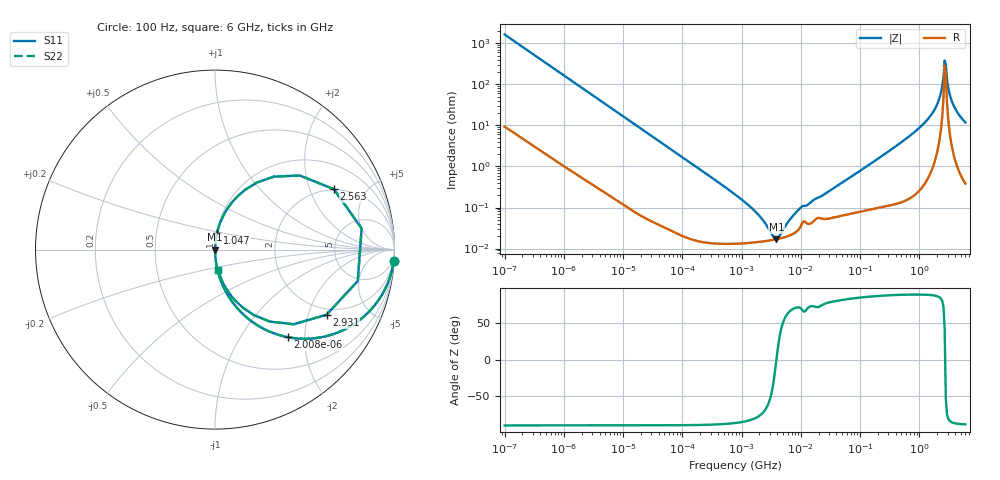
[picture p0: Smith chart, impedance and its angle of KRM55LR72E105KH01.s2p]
!Murata Part Number: KRM55LR72E105KH01
!These Parameters are Measured in Series Mode Connection
!Data Generated on Jan 08, 2026
!  o--ll--o
!Port1  Port2
!  o------o
!Operation Temp=25[degC], DC Bias Voltage=0[V]
!Freq. Start=100[Hz] Stop=6[GHz] 401[Steps]
# Hz S RI R 50
!Freq.(Hz) S11(Real) S11(Imag) S21(Real) S21(Imag) S12(Real) S12(Imag) S22(Real) S22(Imag)
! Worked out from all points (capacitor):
!   401 points, 100 Hz to 6 GHz, reference 50 ohm
!   read as one part in series: C = 972 nF near 109 Hz
!   lowest |Z| = 16.8 mohm at 3.882 MHz (marker M1)
!   series resonance near 3.878 MHz, so ESL is about 1.7 nH
!   S11 on the Smith chart (normalised r, x): 100 Hz: 1, -33; 2.008 kHz: 1.01, -1.65; 1.047 GHz: 1.01, +0.18; 2.563 GHz: 1.97, +2.96; 2.931 GHz: 1.75, -2.64; 6 GHz: 1.01, -0.23
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100  0.9959 -0.0609  0.00407 0.0609  0.00407 0.0609  0.9959 -0.0609
600  0.8813 -0.3204  0.1187 0.3204  0.1187 0.3204  0.8813 -0.3204
1227  0.6429 -0.476  0.3571 0.476  0.3571 0.476  0.6429 -0.476
2008  0.4045 -0.4876  0.5955 0.4876  0.5955 0.4876  0.4045 -0.4876
5882  0.0754 -0.2605  0.9246 0.2605  0.9246 0.2605  0.0754 -0.2605
40335  0.00209 -0.0414  0.9979 0.0414  0.9979 0.0414  0.00209 -0.0414
774597  0.000135 -0.00208  0.9999 0.00208  0.9999 0.00208  0.000135 -0.00208
1813585  0.000144 -0.000716  0.9999 0.000716  0.9999 0.000716  0.000144 -0.000716
3394479  0.000162 -0.000113  0.9998 0.000113  0.9998 0.000113  0.000162 -0.000113
3882480  0.000168 1e-06  0.9998 -1e-06  0.9998 -1e-06  0.000168 1e-06
9090158  0.000287 0.000824  0.9997 -0.000824  0.9997 -0.000824  0.000287 0.000824
1.555665e7  0.000433 0.00137  0.9996 -0.00137  0.9996 -0.00137  0.000433 0.00137
3.124326e8  0.00168 0.0239  0.9983 -0.0239  0.9983 -0.0239  0.00168 0.0239
1.046602e9  0.0111 0.091  0.9889 -0.091  0.9889 -0.091  0.0111 0.091
1.95892e9  0.0987 0.2679  0.9013 -0.2679  0.9013 -0.2679  0.0987 0.2679
2.34314e9  0.3286 0.4068  0.6714 -0.4068  0.6714 -0.4068  0.3286 0.4068
2.562649e9  0.6626 0.3366  0.3374 -0.3366  0.3374 -0.3366  0.6626 0.3366
2.679998e9  0.817 0.1175  0.183 -0.1175  0.183 -0.1175  0.817 0.1175
2.931063e9  0.6213 -0.3631  0.3787 0.3631  0.3787 0.3631  0.6213 -0.3631
3.205649e9  0.3049 -0.4009  0.6951 0.4009  0.6951 0.4009  0.3049 -0.4009
3.666503e9  0.1206 -0.292  0.8794 0.292  0.8794 0.292  0.1206 -0.292
6e9  0.0173 -0.115  0.9827 0.115  0.9827 0.115  0.0173 -0.115
